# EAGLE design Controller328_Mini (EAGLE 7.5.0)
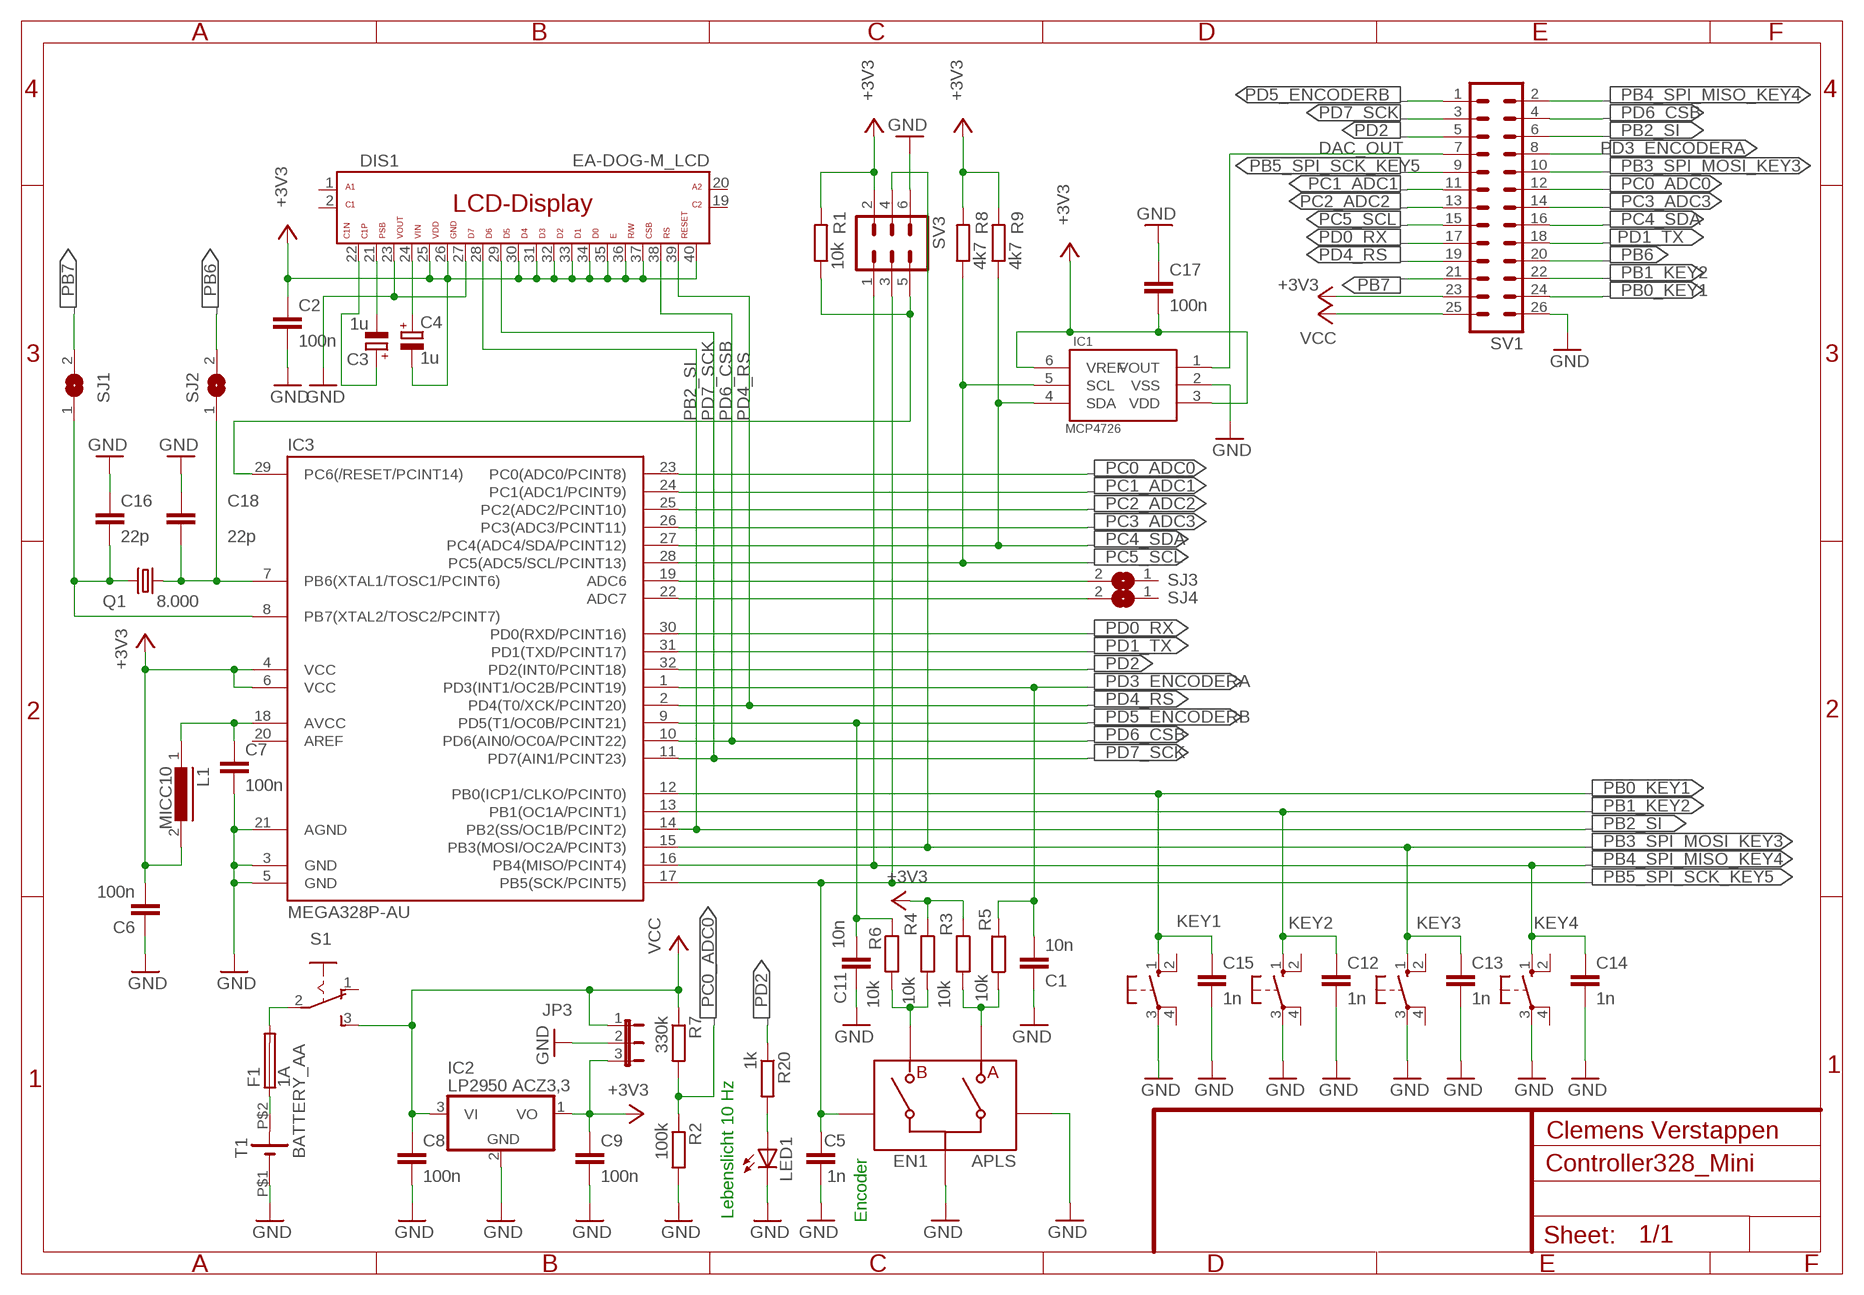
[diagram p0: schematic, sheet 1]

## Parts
C1  10n  C-EU025-024X044  [C025-024X044]
C2  100n  C-EU025-024X044  [C025-024X044]
C3  1u  CPOL-EUE2-5  [E2-5]
C4  1u  CPOL-EUE2-5  [E2-5]
C5  1n  C-EU025-024X044  [C025-024X044]
C6  100n  C-EU025-024X044  [C025-024X044]
C7  100n  C-EU025-024X044  [C025-024X044]
C8  100n  C-EU025-024X044  [C025-024X044]
C9  100n  C-EU025-024X044  [C025-024X044]
C11  10n  C-EU025-024X044  [C025-024X044]
C12  1n  C-EU025-024X044  [C025-024X044]
C13  1n  C-EU025-024X044  [C025-024X044]
C14  1n  C-EU025-024X044  [C025-024X044]
C15  1n  C-EU025-024X044  [C025-024X044]
C16  22p  C-EU025-024X044  [C025-024X044]
C17  100n  C-EU025-024X044  [C025-024X044]
C18  22p  C-EU025-024X044  [C025-024X044]
DIS1  EA-DOG-M_LCD  [EA-DOG-M_LCD]
EN1  APLS  ALPS_ENCODER  [ALPS_ENCODER_EC12]
F1  1A  PICOFUSE  [PICOFUSE]
IC1  MCP4726  [SOT23-6]
IC2  LP2950 ACZ3,3  78L05Z  [TO92]
IC3  MEGA328P-AU  MEGA48/88/168-AU  [TQFP32-08]
JP3  JP2E  [JP2]
KEY1  10-XX  [B3F-10XX]
KEY2  10-XX  [B3F-10XX]
KEY3  10-XX  [B3F-10XX]
KEY4  10-XX  [B3F-10XX]
L1  MICC10  [MICC10]
LED1  LED5MM  [LED5MM]
Q1  8.000  CRYTALHC49U-V  [HC49U-V]
R1  10k  R-EU_0204/7  [0204/7]
R2  100k  R-EU_0204/7  [0204/7]
R3  10k  R-EU_0204/7  [0204/7]
R4  10k  R-EU_0204/7  [0204/7]
R5  10k  R-EU_0204/7  [0204/7]
R6  10k  R-EU_0204/7  [0204/7]
R7  330k  R-EU_0204/7  [0204/7]
R8  4k7  R-EU_0204/7  [0204/7]
R9  4k7  R-EU_0204/7  [0204/7]
R20  1k  R-EU_0204/7  [0204/7]
S1  M251  [M251]
SJ1  SJW  [SJW]
SJ2  SJW  [SJW]
SJ3  SJW  [SJW]
SJ4  SJW  [SJW]
SV1  ML26L  [ML26L]
SV3  ML6  [ML6]
T1  BATTERY_AA  [BATTERIEHALTER_MIGNON]

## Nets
+3V3: C2.1 C4.- C6.2 C9.1 C17.2 DIS1.25 DIS1.26 DIS1.30 DIS1.31 DIS1.32 DIS1.33 DIS1.34 DIS1.35 DIS1.36 DIS1.37 DIS1.40 IC1.3(VDD) IC1.6(VREF) IC2.1(VO) IC3.4(VCC) IC3.6(VCC) JP3.3 L1.2 R1.2 R3.1 R4.1 R8.2 R9.2 SV1.23 SV3.2
DAC_OUT: IC1.1(VOUT) SV1.7
GND: C1.1 C2.2 C5.2 C6.1 C7.2 C8.2 C9.2 C11.1 C12.2 C13.2 C14.2 C15.2 C16.1 C17.1 C18.1 DIS1.23 DIS1.27 EN1.C EN1.D IC1.2(VSS) IC2.2(GND) IC3.3(GND) IC3.5(GND) IC3.21(AGND) JP3.2 KEY1.3(P) KEY2.3(P) KEY3.3(P) KEY4.3(P) LED1.K(C) R2.2 SV1.26 SV3.6 T1.P$1(-)
N$1: EN1.A R3.2 R5.1
N$2: IC3.19(ADC6) SJ3.2
N$3: LED1.A R20.2
N$4: IC3.22(ADC7) SJ4.2
N$10: F1.1 T1.P$2(+)
N$11: C7.1 IC3.18(AVCC) L1.1
N$12: F1.2 S1.2(P)
N$22: C3.+ DIS1.22
N$23: C3.- DIS1.21
N$24: C4.+ DIS1.24
N$44: EN1.B R4.2 R6.2
PB0_KEY1: C15.1 IC3.12(PB0(ICP1/CLKO/PCINT0)) KEY1.1(S) SV1.24
PB1_KEY2: C12.1 IC3.13(PB1(OC1A/PCINT1)) KEY2.1(S) SV1.22
PB2_SI: DIS1.28 IC3.14(PB2(SS/OC1B/PCINT2)) SV1.6
PB3_SPI_MOSI_KEY3: C13.1 IC3.15(PB3(MOSI/OC2A/PCINT3)) KEY3.1(S) SV1.10 SV3.4
PB4_SPI_MISO_KEY4: C14.1 IC3.16(PB4(MISO/PCINT4)) KEY4.1(S) SV1.2 SV3.1
PB5_SPI_SCK_KEY5: C5.1 EN1.E IC3.17(PB5(SCK/PCINT5)) SV1.9 SV3.3
PB6: SJ2.2 SV1.20
PB6_XTAL1: C18.2 IC3.7(PB6(XTAL1/TOSC1/PCINT6)) Q1.1 SJ2.1
PB7: SJ1.2 SV1.21
PB7_XTAL2: C16.2 IC3.8(PB7(XTAL2/TOSC2/PCINT7)) Q1.2 SJ1.1
PC0_ADC0: IC3.23(PC0(ADC0/PCINT8)) R2.1 R7.2 SV1.12
PC1_ADC1: IC3.24(PC1(ADC1/PCINT9)) SV1.11
PC2_ADC2: IC3.25(PC2(ADC2/PCINT10)) SV1.13
PC3_ADC3: IC3.26(PC3(ADC3/PCINT11)) SV1.14
PC4_SDA: IC1.4(SDA) IC3.27(PC4(ADC4/SDA/PCINT12)) R9.1 SV1.16
PC5_SCL: IC1.5(SCL) IC3.28(PC5(ADC5/SCL/PCINT13)) R8.1 SV1.15
PC6_RST: IC3.29(PC6(/RESET/PCINT14)) R1.1 SV3.5
PD0_RX: IC3.30(PD0(RXD/PCINT16)) SV1.17
PD1_TX: IC3.31(PD1(TXD/PCINT17)) SV1.18
PD2: IC3.32(PD2(INT0/PCINT18)) R20.1 SV1.5
PD3_ENCODERA: C1.2 IC3.1(PD3(INT1/OC2B/PCINT19)) R5.2 SV1.8
PD4_RS: DIS1.39 IC3.2(PD4(T0/XCK/PCINT20)) SV1.19
PD5_ENCODERB: C11.2 IC3.9(PD5(T1/OC0B/PCINT21)) R6.1 SV1.1
PD6_CSB: DIS1.38 IC3.10(PD6(AIN0/OC0A/PCINT22)) SV1.4
PD7_SCK: DIS1.29 IC3.11(PD7(AIN1/PCINT23)) SV1.3
VCC: C8.1 IC2.3(VI) JP3.1 R7.1 S1.3(S) SV1.25
Unconnected: DIS1.1 DIS1.2 DIS1.19 DIS1.20 IC3.20(AREF) KEY1.2(S1) KEY1.4(P1) KEY2.2(S1) KEY2.4(P1) KEY3.2(S1) KEY3.4(P1) KEY4.2(S1) KEY4.4(P1) S1.1(O) SJ3.1 SJ4.1

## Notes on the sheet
- Clemens Verstappen
- Encoder
- Lebenslicht 10 Hz

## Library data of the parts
C1 C2 C5-C9 C11-C18 = rcl:C-EU: CAPACITOR, European symbol
C3 C4 = rcl:CPOL-EU: POLARIZED CAPACITOR, European symbol
DIS1 = 1_USER:EA-DOG-M_LCD
EN1 = TEWE:ALPS_ENCODER
F1 = fuse:PICOFUSE: PICOFUSE
IC1 = TEWE:MCP4726
IC2 = linear:78*: Positive VOLTAGE REGULATOR
IC3 = avr-4:MEGA48/88/168
JP3 = jumper:JP2E: JUMPER
KEY1-KEY4 = switch-omron:10-XX: OMRON SWITCH
L1 = inductors:MICC10: INDUCTOR
LED1 = led:LED: LED
Q1 = crystal:CRYTAL: CRYSTAL
R1-R9 R20 = rcl:R-EU_: RESISTOR, European symbol
S1 = switch:M251: SLIDING SWITCH Mors, distributor Buerklin, 11G702
SJ1-SJ4 = jumper:SJ: SMD solder JUMPER
SV1 = con-harting-ml:ML26: HARTING
SV3 = con-harting-ml:ML6: HARTING
T1 = TEWE:BATTERY_AA

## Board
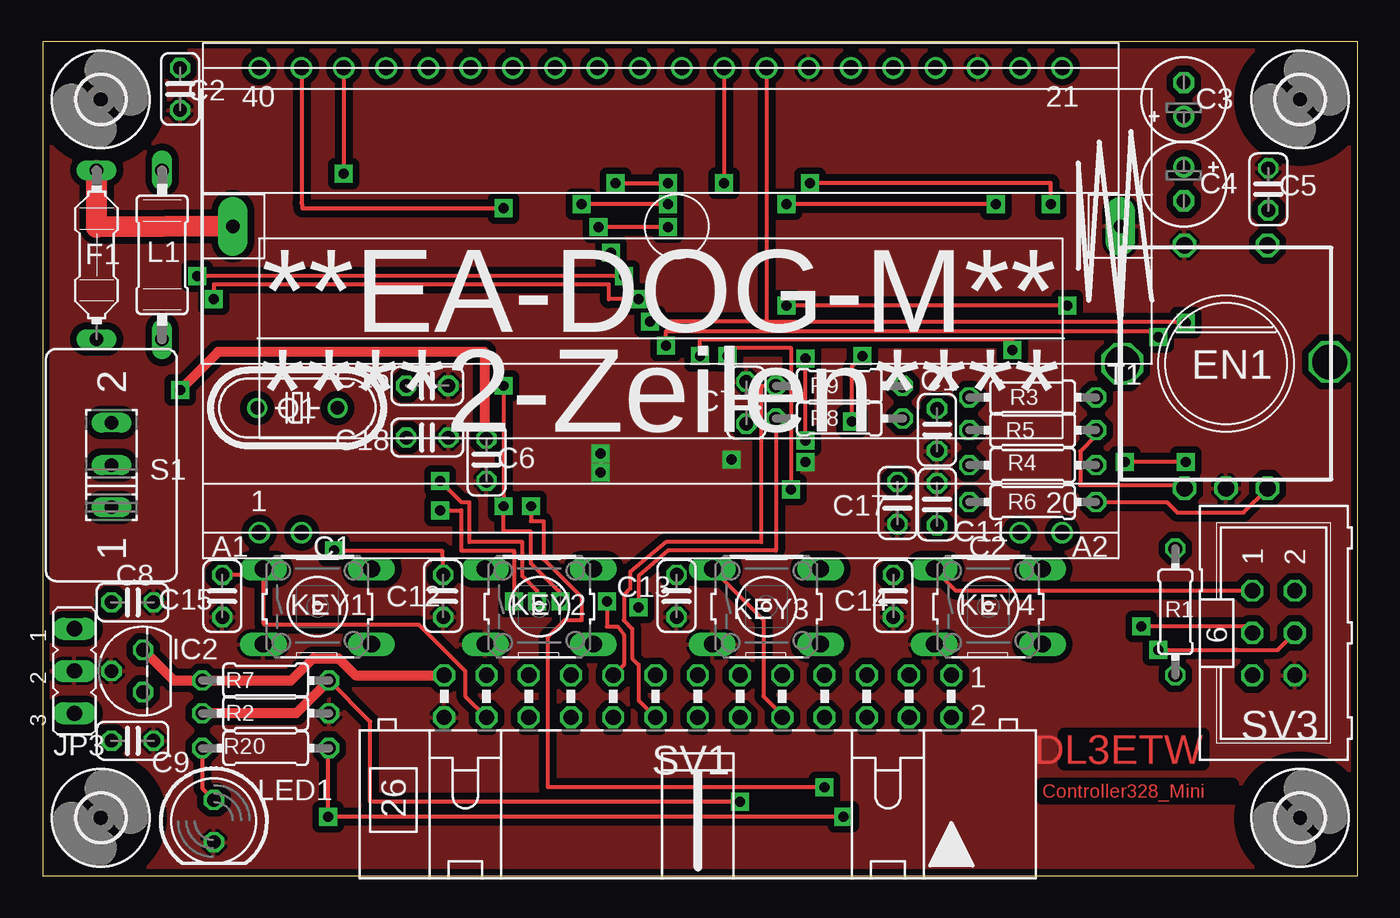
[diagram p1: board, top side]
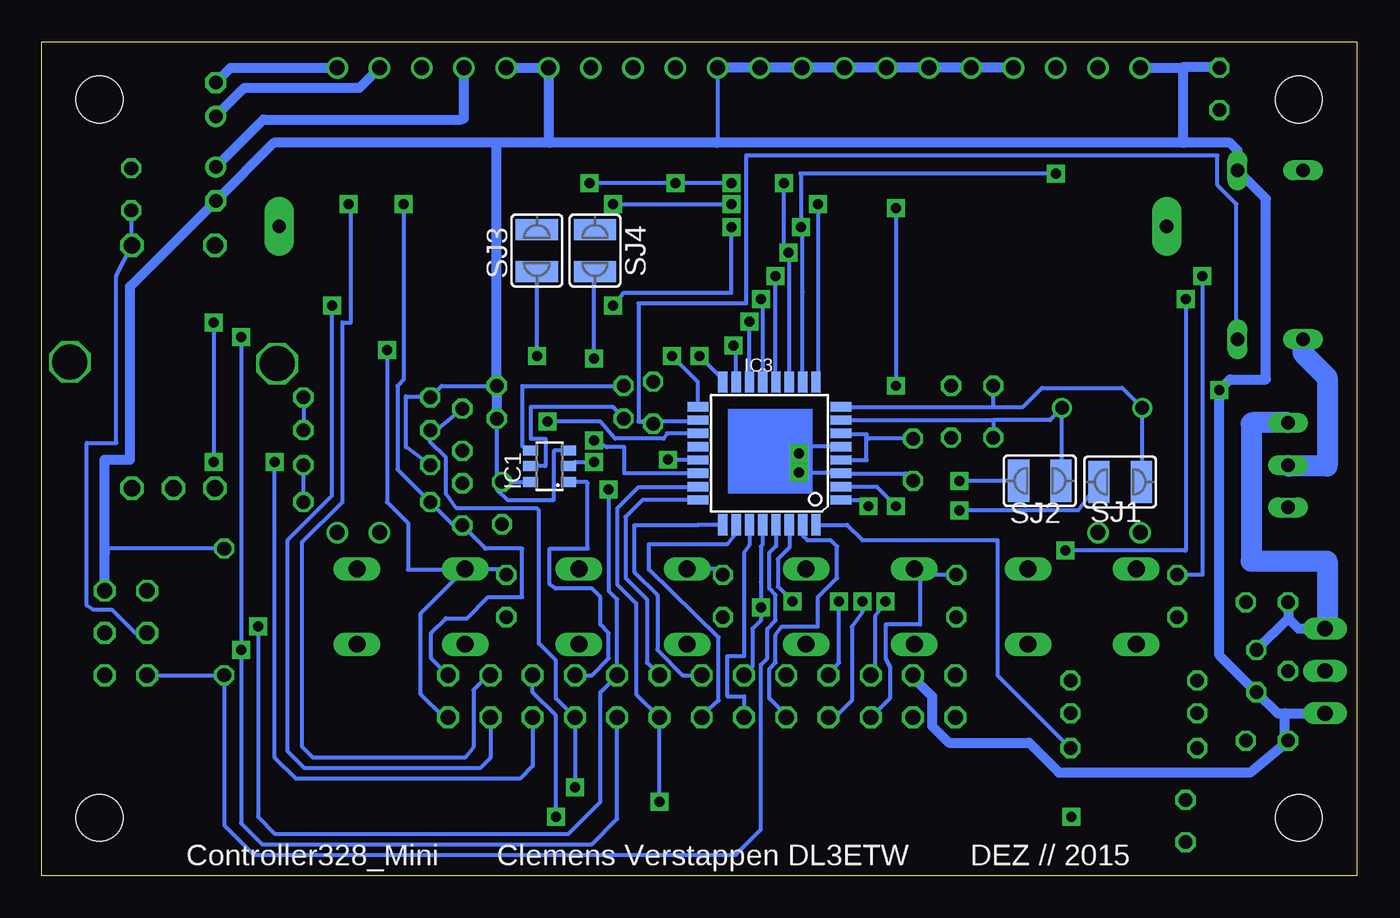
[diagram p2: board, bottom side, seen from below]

Size 79.05 x 50.16 mm. Coordinates in mm from the lower left corner, seen from the top.
Outline: 0,0 79.05,0 79.05,50.16 0,50.16 0,0
Copper layers (1*16): Top 0.035mm / dielectric 1.5mm / Bottom 0.035mm
Design rules "PCB-POOL Standard": minimum track width 0.15mm, minimum drill 0.3mm, track to track 0.15mm, track to pad 0.15mm, pad to pad 0.15mm, via to via 0.15mm, smd to smd 0.15mm, copper to edge 0.3mm, drill to drill 0.2mm, minimum pad ring 0.2mm, minimum via ring 0.15mm, stop-mask expansion 0.075mm, vias tented up to drill 0mil, thermal gap 0.2mm

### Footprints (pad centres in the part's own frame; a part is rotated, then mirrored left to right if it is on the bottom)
C025-024X044 = drill 0.813 octagon: 1 -1.27,0; 2 1.27,0
E2-5 = drill 0.813 pad 1.27: + -1.016,0 | drill 0.813 pad 1.27 octagon: - 1.016,0
EA-DOG-M_LCD = drill 0.9: 1 -24.13,-27.94; 2 -21.59,-27.94; 19 21.59,-27.94; 20 24.13,-27.94; 21 24.13,0; 22 21.59,0; 23 19.05,0; 24 16.51,0; 25 13.97,0; 26 11.43,0; 27 8.89,0; 28 6.35,0; 29 3.81,0; 30 1.27,0; 31 -1.27,0; 32 -3.81,0; 33 -6.35,0; 34 -8.89,0; 35 -11.43,0; 36 -13.97,0; 37 -16.51,0; 38 -19.05,0; 39 -21.59,0; 40 -24.13,0
ALPS_ENCODER_EC12 = drill 2.1 octagon: 1 -6.23,0; 2 6.23,0.1 | drill 1 octagon: A -2.5,-7.5; B 2.5,-7.5; C 0,-7.5; D -2.5,7.105; E 2.5,7.105
PICOFUSE = drill 0.813 long: 1 -5.08,0; 2 5.08,0
SOT23-6 = smd 0.6 x 0.9: 1 -0.95,-1.15; 2 0,-1.15; 3 0.95,-1.15; 4 0.95,1.15; 5 0,1.15; 6 -0.95,1.15
TO92 = drill 0.813 octagon: 1 -1.27,0; 2 0,1.905; 3 1.27,0
TQFP32-08 = smd 1.27 x 0.559: 1 -4.293,2.8; 2 -4.293,2; 3 -4.293,1.2; 4 -4.293,0.4; 5 -4.293,-0.4; 6 -4.293,-1.2; 7 -4.293,-2; 8 -4.293,-2.8; 17 4.293,-2.8; 18 4.293,-2; 19 4.293,-1.2; 20 4.293,-0.4; 21 4.293,0.4; 22 4.293,1.2; 23 4.293,2; 24 4.293,2.8 | smd 0.559 x 1.27: 9 -2.8,-4.293; 10 -2,-4.293; 11 -1.2,-4.293; 12 -0.4,-4.293; 13 0.4,-4.293; 14 1.2,-4.293; 15 2,-4.293; 16 2.8,-4.293; 25 2.8,4.293; 26 2,4.293; 27 1.2,4.293; 28 0.4,4.293; 29 -0.4,4.293; 30 -1.2,4.293; 31 -2,4.293; 32 -2.8,4.293
JP2 = drill 0.914 long: 1 -2.54,0; 2 0,0; 3 2.54,0
B3F-10XX = drill 1.016 long: 1 -3.251,2.261; 2 3.251,2.261; 3 -3.251,-2.261; 4 3.251,-2.261
MICC10 = drill 0.813 long: 1 -5.08,0; 2 5.08,0
LED5MM = drill 0.813 octagon: A -1.27,0; K 1.27,0
HC49U-V = drill 0.813: 1 -2.413,0; 2 2.413,0
0204/7 = drill 0.813 octagon: 1 -3.81,0; 2 3.81,0
M251 = drill 0.813 long: 1 -2.54,0; 2 0,0; 3 2.54,0
SJW = smd 1.27 x 2.54: 1 -1.27,0; 2 1.27,0
ML26L = drill 0.914 octagon: 1 -15.24,-1.27; 2 -15.24,1.27; 3 -12.7,-1.27; 4 -12.7,1.27; 5 -10.16,-1.27; 6 -10.16,1.27; 7 -7.62,-1.27; 8 -7.62,1.27; 9 -5.08,-1.27; 10 -5.08,1.27; 11 -2.54,-1.27; 12 -2.54,1.27; 13 0,-1.27; 14 0,1.27; 15 2.54,-1.27; 16 2.54,1.27; 17 5.08,-1.27; 18 5.08,1.27; 19 7.62,-1.27; 20 7.62,1.27; 21 10.16,-1.27; 22 10.16,1.27; 23 12.7,-1.27; 24 12.7,1.27; 25 15.24,-1.27; 26 15.24,1.27
ML6 = drill 0.914 octagon: 1 -2.54,-1.27; 2 -2.54,1.27; 3 0,-1.27; 4 0,1.27; 5 2.54,-1.27; 6 2.54,1.27
BATTERIEHALTER_MIGNON = drill 0.8 pad 1.778 long: P$1 -26.67,0; P$2 26.67,0
2,8 = hole 2.8: 0,0

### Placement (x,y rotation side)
C1  53.76,26.82 90 top
C2  8.26,47.31 270 top
C3  68.58,46.67 90 top
C4  68.58,41.59 270 top
C5  73.66,41.27 90 top
C6  26.67,25.02 90 top
C7  42.29,28.45 90 top
C8  5.4,16.45 0 top
C9  5.4,8.13 0 top
C11  53.75,22.34 270 top
C12  24.07,16.83 270 top
C13  38.1,16.83 270 top
C14  51.12,16.83 270 top
C15  10.79,16.83 270 top
C16  23.11,29.47 180 top
C17  51.37,22.42 90 top
C18  23.12,26.35 180 top
DIS1  37.15,48.58 0 top
EN1  71.12,30.8 0 top
F1  3.24,37.34 270 top
IC1  48.51,24.64 90 bottom
IC2  6.03,12.32 90 top
IC3  35.3,25.4 180 bottom
JP3  1.91,12.32 270 top
KEY1  16.51,16.19 0 top
KEY2  29.84,16.19 0 top
KEY3  43.5,16.19 0 top
KEY4  56.83,16.19 0 top
L1  7.18,37.34 90 top
LED1  10.29,3.3 270 top
Q1  15.3,28.13 180 top
R1  68.07,15.88 90 top
R2  13.4,9.78 0 top
R3  59.5,28.77 0 top
R4  59.5,24.7 0 top
R5  59.5,26.8 180 top
R6  59.5,22.48 0 top
R7  13.4,11.75 0 top
R8  47.88,27.5 0 top
R9  47.88,29.46 0 top
R20  13.4,7.68 180 top
S1  4.13,24.7 90 top
SJ1  14.22,23.69 180 bottom
SJ2  19.05,23.75 180 bottom
SJ3  49.28,37.59 270 bottom
SJ4  45.78,37.59 270 bottom
SV1  39.37,10.79 180 top
SV3  73.98,14.61 270 top
T1  38.1,39.05 180 top
U$4  [2,8]  3.49,46.67 0 top
U$5  [2,8]  75.56,46.67 0 top
U$10  [2,8]  3.49,3.49 0 top
U$13  [2,8]  75.56,3.49 0 top

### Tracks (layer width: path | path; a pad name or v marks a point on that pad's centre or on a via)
+3V3  (via drill 0.6)
  Top 0.61: C6.2 26.54,26.42 26.54,31.5 10.54,31.5 v8.26,29.21
  Bottom 0.254: IC3.4 29.46,25 29.46,26.42 | 29.46,26.42 29.46,26.54 31.01,26.54 IC3.6 | R4.1 57.15,25.78 57.15,28.83 55.69,28.83 R3.1 54.99,29.46 R9.2 | R8.2 51.69,23.62 | 51.69,23.62 C17.2 50.99,23.69 IC1.6 | 51.69,23.62 51.69,23.24 51.05,22.61 48.26,22.61 48.26,25.53 48.19,25.59 IC1.3 | R1.2 74.99,19.68 75.25,19.43 | C6.2 29.34,26.29 29.46,26.42 | DIS1.30 38.42,44.13
  Bottom 0.61: 4.32,9.78 4.76,9.78 IC2.1 8.26,13.27 v8.26,29.21 7.62,29.84 5.46,29.84 5.46,40.7 L1.2 7.18,43.62 7.62,44.07 10.41,44.07 | 4.32,9.78 JP3.3 | 4.32,9.78 4.32,8.32 C9.1 6.41,6.22 17.91,6.22 19.68,8 24.51,8 25.53,9.02 25.53,10.79 26.67,11.94 SV1.23 | 10.41,44.07 10.41,48.58 | C2.1 8.26,48.64 10.41,48.64 10.41,48.58 | DIS1.40 10.41,48.58 | 10.41,44.07 38.48,44.07 | 38.48,44.07 48.51,44.07 | 48.51,44.07 51.69,44.07 | 51.69,44.07 65.09,44.07 C4.- 73.72,35.43 73.72,25.02 75.25,25.02 75.25,19.68 75.25,19.43 SV3.2 | DIS1.37 DIS1.36 DIS1.35 DIS1.34 DIS1.33 DIS1.32 DIS1.31 DIS1.30 | 38.42,44.13 38.48,44.07 | 48.51,44.07 48.58,44.13 DIS1.26 DIS1.25 | 51.69,44.07 R9.2 R8.2
DAC_OUT
  Bottom 0.254: SV1.7 45.97,12.06 44.96,13.08 44.96,14.61 45.47,15.11 45.47,16.76 45.97,17.27 48.13,17.27 48.51,17.53 48.51,19.68 46.23,19.68 46.23,23.62 46.3,23.69 IC1.1
GND  (via drill 0.6)
  Top 0.254: v33.53,25.4 v33.53,24.26
  Bottom 0.254: IC3.21 41.38,25 v41.4,25.02 | IC3.5 33.13,25.8 v33.53,25.4 | v33.53,24.26 31.07,24.26 IC3.3 27.12,24.2 C6.1 | IC1.2 arc-90 46.98,24.89 v45.85,24.89
  pour Top (isolate 0.406): 0.13,0.13 0.13,50.04 78.87,50.04 78.87,0.13
N$1
  Top 0.254: R5.1 63.31,26.48 62.36,25.53 62.36,23.5 68.42,23.5 EN1.A
  Bottom 0.254: R3.2 R5.1
N$2  (via drill 0.6)
  Top 0.254: v48.64,27.3 48.64,30.61 v49.28,31.24
  Bottom 0.254: IC3.19 41.47,26.6 41.66,26.29 44.58,26.29 45.47,27.3 v48.64,27.3 | v49.28,31.24 SJ3.2
N$3
  Top 0.254: R20.2 9.59,5.27 LED1.A
N$4  (via drill 0.6)
  Top 0.254: v45.85,26.16 v45.85,31.11
  Bottom 0.254: IC3.22 44.01,24.2 44.02,25.78 45.09,25.78 v45.85,26.16 | v45.85,31.11 45.85,36.26 SJ4.2
N$10
  Top 1.27: T1.P$2 3.24,38.99 F1.1
N$11
  Bottom 0.254: L1.1 7.24,32.32 7.24,40.39 8.38,41.53 8.38,43.31 36.7,43.31 36.7,34.42 43.18,34.42 43.18,27.3 | 43.18,27.3 41.91,27.18 C7.1 | IC3.18 39.6,27.3 43.18,27.3
N$12
  Bottom 1.27: F1.2 3.24,31.43 1.78,29.97 1.78,24.64 4.06,24.64 S1.2
N$22
  Bottom 0.61: C3.+ 66.86,47.37 59.94,47.37 DIS1.22
N$23
  Bottom 0.61: C3.- 67.69,48.58 DIS1.21
N$24
  Bottom 0.61: C4.+ 65.72,45.47 53.85,45.47 53.66,45.53 DIS1.24
N$44
  Top 0.254: R6.2 67.56,22.48 68.2,21.84 72.17,21.84 EN1.B
  Bottom 0.254: R6.2 R4.2
PB0_KEY1  (via drill 0.6)
  Top 0.254: C15.1 12.9,18.1 KEY1.1 13.26,15.19 13.34,15.11 22.61,15.11 25.4,12.32 25.4,10.79 SV1.24 | v34.92,36.07 v9.27,36.07
  Bottom 0.254: v9.27,36.07 9.27,18.1 C15.1 | IC3.12 34.92,29.84 v34.92,36.07
PB1_KEY2  (via drill 0.6)
  Top 0.254: v35.81,34.67 34.04,34.67 34.04,35.56 10.29,35.56 v10.29,34.67 | v17.53,19.56 24,19.56 C12.1
  Bottom 0.254: IC3.13 35.69,29.58 35.69,34.67 v35.81,34.67 | v10.29,34.67 10.29,19.56 v17.53,19.56 | C12.1 26.24,18.1 | 26.24,18.1 KEY2.1 | 26.24,18.1 26.25,17.4 26.24,15.11 28.32,15.11 28.32,13.08 28.07,12.57 28.07,10.67 SV1.22
PB2_SI  (via drill 0.6)
  Top 0.254: DIS1.28 43.5,33.33 | 43.5,33.33 v36.5,33.33 | 43.5,33.33 68.65,33.33 v68.71,33.27 | v68.71,24.89 v65.02,24.89
  Bottom 0.254: IC3.14 v36.5,33.33 | SV1.6 49.53,6.6 50.29,5.84 63.75,5.84 65.02,7.11 v65.02,24.89 | v68.71,33.27 v68.71,24.89
PB3_SPI_MOSI_KEY3  (via drill 0.6)
  Top 0.254: v67.06,13.59 71.75,13.59 72.96,13.59 74.23,13.59 SV3.4 | v37.47,31.88 37.47,32.77 67.06,32.77 v67.06,32.38 | KEY3.1 43.31,15.39 43.31,10.79 44.45,9.65 SV1.10
  Bottom 0.254: IC3.15 37.3,31.72 v37.47,31.88 | v67.06,32.38 v67.06,13.59 67.06,3.17 65.79,1.91 45.97,1.91 44.45,3.43 SV1.10 | C13.1 38.46,18.45 KEY3.1
PB4_SPI_MISO_KEY4  (via drill 0.6)
  Top 0.254: v39.5,31.24 39.5,32.26 58.29,32.26 v58.29,31.62 | SV3.1 54.89,17.14 KEY4.1
  Bottom 0.254: IC3.16 38.1,29.85 v39.5,31.24 | v58.29,31.62 58.29,22.48 57.02,21.21 57.02,18.41 53.62,18.41 | C14.1 51.47,18.45 KEY4.1 53.62,18.41 | SV1.2 54.86,9.53 56.26,10.92 56.26,15.77 53.62,18.41
PB5_SPI_SCK_KEY5  (via drill 0.6)
  Top 0.254: v41.15,31.24 41.15,31.75 44.96,31.75 v44.96,23.24 | SV3.3 72.26,14.99 v66.04,14.99
  Bottom 0.254: IC3.17 39.6,29.69 v41.15,31.24 | v44.96,23.24 44.96,17.14 44.45,16.64 SV1.9 45.47,11.05 45.47,4.45 47.37,2.54 65.02,2.54 66.04,3.56 v66.04,14.99 | C5.1 73.62,39.97 EN1.E 74.55,36.08 74.55,26.04 76.33,26.04 76.33,16.26 75.95,16 74.8,16 73.41,14.61 SV3.3
PB6  (via drill 0.6)
  Top 0.254: v29.72,16.51 29.72,17.14 28.83,18.03 28.83,20.07 25.65,20.07 25.65,22.48 25.15,22.48 v23.88,23.75
  Bottom 0.254: v29.72,16.51 29.72,15.88 30.35,14.99 30.35,10.54 31.37,9.53 SV1.20 | SJ2.2 v23.88,23.75
PB6_XTAL1
  Bottom 0.254: 30.73,27.43 IC3.7 21.85,27.4 | 21.85,27.4 C18.2 | 21.85,27.4 18.45,27.4 Q1.1 17.72,23.81 SJ2.1
PB7  (via drill 0.6)
  Top 0.254: v28.32,16.51 28.32,19.56 25.15,19.56 25.15,21.97 v23.88,21.97
  Bottom 0.254: v28.32,16.51 28.96,15.62 28.96,12.32 SV1.21 | SJ1.2 16.76,21.97 v23.88,21.97
PB7_XTAL2
  Bottom 0.254: IC3.8 21.84,28.2 | 21.84,28.2 C16.2 | 21.84,28.2 20.06,28.2 18.92,29.34 14.1,29.34 Q1.2 12.89,23.75 SJ1.1
PC0_ADC0  (via drill 0.6)
  Top 0.254: v41.91,4.45 19.68,4.45 19.68,9.27 R7.2 | 15.11,9.65 14.99,9.78
  Top 0.61: R7.2 15.24,9.78 14.99,9.78 R2.1
  Bottom 0.254: v41.91,4.45 SV1.12 43.31,10.92 43.31,16.38 44.45,17.53 44.45,22.1 43.18,23.37 39.6,23.37 IC3.23
PC1_ADC1
  Bottom 0.254: IC3.24 41.27,22.6 41.28,22.61 42.93,22.61 43.95,21.59 43.94,17.91 42.67,16.64 42.67,12.83 SV1.11
PC2_ADC2
  Bottom 0.254: IC3.25 39.6,21.11 39.62,21.08 43.43,21.08 43.43,18.29 42.04,16.89 42.04,13.59 40.51,12.06 SV1.13
PC3_ADC3
  Bottom 0.254: IC3.26 37.3,20.61 37.85,19.94 42.55,19.94 42.55,18.41 38.35,14.35 38.35,10.54 39.37,9.65 SV1.14
PC4_SDA
  Top 0.254: R9.1 43.18,29.46 43.18,20.07 37.47,20.07 35.31,18.29 35.31,17.27 34.92,16.89 34.92,15.37 35.43,14.86 35.43,13.08 35.81,12.7 35.81,10.54 SV1.16
  Bottom 0.254: IC3.27 36.5,19.88 36.83,19.43 36.83,13.21 37.85,13.21 37.85,10.79 36.83,10.79 SV1.16 | R9.1 50.16,29.46 50.16,25.84 IC1.4
PC5_SCL  (via drill 0.6)
  Top 0.254: R8.1 44.07,19.56 37.59,19.56 35.81,18.03 v35.81,16.13 | v35.81,16.13
  Bottom 0.254: IC3.28 35.71,19.93 35.81,19.78 35.81,17.65 v35.81,16.13 35.81,15.37 36.32,14.86 36.32,12.57 SV1.15 | R8.1 44.64,28.13 44.7,28.19 49.66,28.19 49.66,26.29 48.77,26.29 48.77,24.64 IC1.5
PC6_RST
  Bottom 0.254: IC3.29 34.9,19.83 35.31,19.43 35.31,17.27 34.92,16.89 34.92,15.37 35.43,14.86 35.43,13.08 35.81,12.7 35.81,2.79 37.34,1.27 66.29,1.27 68.07,3.05 R1.1 SV3.5 72.77,12
PD0_RX  (via drill 0.6)
  Top 0.254: v33.91,16.51 33.91,14.99 34.54,14.99 34.92,14.48 34.92,12.7 SV1.17
  Bottom 0.254: IC3.30 34.1,19.74 34.8,19.05 34.8,17.4 v33.91,16.51
PD1_TX
  Bottom 0.254: IC3.31 33.3,20.48 33.02,20.19 31.62,20.19 31.24,19.81 31.24,17.91 32.38,16.76 32.38,14.99 34.54,14.99 34.92,14.48 34.92,12.83 35.31,12.45 35.31,10.67 34.16,9.53 SV1.18
PD2  (via drill 0.6)
  Top 0.254: v48.13,3.56 v17.14,3.56 17.14,7.62 R20.1
  Bottom 0.254: IC3.32 30.63,21.11 29.72,20.19 21.59,20.19 21.59,12.06 R20.1 17.14,7.62 | v48.13,3.56 48.13,9.65 49.53,11.05 SV1.5
PD3_ENCODERA  (via drill 0.6)
  Top 0.254: v29.34,22.23 29.34,21.34 30.1,21.34 30.1,19.05 32.38,16.76 32.38,15.37 31.37,15.37 30.35,14.35 30.35,5.46 | 30.35,5.46 30.35,5.33 | v46.99,5.33 30.48,5.33 30.35,5.46
  Bottom 0.254: C1.2 55.31,26.8 R5.2 55.69,26.1 54.74,25.15 54.74,22.99 54.1,22.1 49.28,22.1 49.15,21.97 49.15,13.97 48.13,12.95 48.13,10.67 SV1.8 v46.99,5.33 | IC3.1 29.71,22.6 v29.34,22.23
PD4_RS  (via drill 0.6)
  Top 0.254: DIS1.39 15.56,40.45 15.62,40.13 v27.69,40.13 | v27.69,29.46 v27.69,22.23 27.69,20.7 29.34,20.7 29.34,18.8 31.11,17.02 v31.11,16.51
  Bottom 0.254: IC3.2 28.86,23.4 v27.69,22.23 | v27.69,40.13 v27.69,29.46 | SV1.19 31.11,12.83 v31.11,16.51
PD5_ENCODERB  (via drill 0.6)
  Top 0.254: v57.28,40.39 v44.7,40.39 | v37.59,40.39 v32.38,40.39
  Bottom 0.254: 32.51,29.7 IC3.9 32.38,29.81 v32.38,40.39 | SV1.1 55.63,13.08 55.63,14.61 54.74,15.49 53.47,15.49 52.2,16.76 50.16,16.76 50.16,19.68 52.37,19.68 C11.2 54.28,21.07 R6.1 57.66,24.45 57.66,29.46 57.28,29.84 v57.28,40.39 | v44.7,40.39 v37.59,40.39
PD6_CSB  (via drill 0.6)
  Top 0.254: v61.59,34.29 v44.7,34.29 | v37.59,38.99 v33.4,38.99 33.27,39.12 | DIS1.38 v18.1,42.23
  Bottom 0.254: IC3.10 33.3,35.08 33.3,39 v33.4,38.99 33.4,42.16 33.47,42.23 v18.1,42.23 | SV1.4 52.07,7.11 52.7,6.48 63.25,6.48 64.26,7.49 64.26,20.19 61.59,22.86 v61.59,34.29 | v44.7,34.29 44.58,34.29 44.07,35.05 37.59,35.05 v37.59,38.99
PD7_SCK  (via drill 0.6)
  Top 0.254: v60.58,40.39 60.58,41.66 v46.1,41.66 | DIS1.29 v40.96,41.66 | v34.42,41.66 v37.59,41.66
  Bottom 0.254: IC3.11 34.1,37.41 v34.16,37.47 34.42,37.72 v34.42,41.66 | SV1.3 52.2,12.06 53.09,11.18 53.09,7.75 53.59,7.11 62.74,7.11 63.37,7.75 63.37,20.07 60.96,22.48 60.96,33.27 60.45,33.27 60.45,40.26 v60.58,40.39 | v46.1,41.66 v40.96,41.66 v37.59,41.66
VCC
  Top 0.61: IC2.3 7.87,11.75 R7.1 14.92,11.75 16.26,13.08 17.78,13.08 18.8,12.06 SV1.25
  Bottom 0.61: C8.1 4.13,15.49 | 4.13,15.49 IC2.3 | JP3.1 3.49,14.86 4.13,15.49
  Bottom 1.27: S1.3 6.29,27.24 6.35,27.18 6.35,18.92 1.78,18.92 1.78,14.99 JP3.1
(copper drawn outside any net)
  shapes: Bottom area x1

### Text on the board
Top: DL3ETW | Controller328_Mini
bNames: DEZ // 2015 | Clemens Verstappen DL3ETW | Controller328_Mini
